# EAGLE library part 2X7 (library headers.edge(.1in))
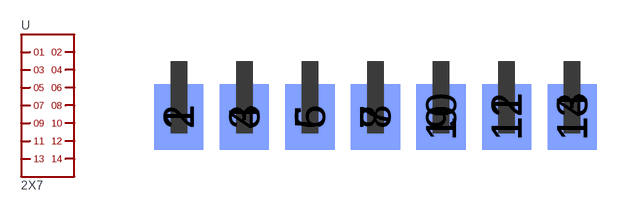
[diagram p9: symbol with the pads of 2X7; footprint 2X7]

Designator prefix -

## 2X7  [2X7]
1  1
2  2
3  3
4  4
5  5
6  6
7  7
8  8
9  9
10  10
11  11
12  12
13  13
14  14

## Footprint 2X7 (pad centres in mm)
smd 1.905 x 2.54: 1 0,-2.159; 3 2.54,-2.159; 5 5.08,-2.159; 7 7.62,-2.159; 9 10.16,-2.159; 11 12.7,-2.159; 13 15.24,-2.159
smd 1.905 x 2.54 bottom: 2 0,-2.159; 4 2.54,-2.159; 6 5.08,-2.159; 8 7.62,-2.159; 10 10.16,-2.159; 12 12.7,-2.159; 14 15.24,-2.159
